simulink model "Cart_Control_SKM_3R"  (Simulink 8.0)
settings: Solver=FixedStepDiscrete  SolverMode=SingleTasking  StartTime=0  StopTime=6  FixedStep=dt  RelTol=1e-3  SampleTimeConstraint=Specified
InitFcn:
  | % Sampling Times %
  | dt0=0.001; dt1=0.01; samples=10;
  | D2R=pi/180;
undefined symbols (not defined in the file or in its folder): DiscIntNeverNeededParam, Volts
libraries: simulink_extras x4, speedgoatlib_IO311 x3, simulink x3, speedgoatlib_IO101 x2, xpclib x1

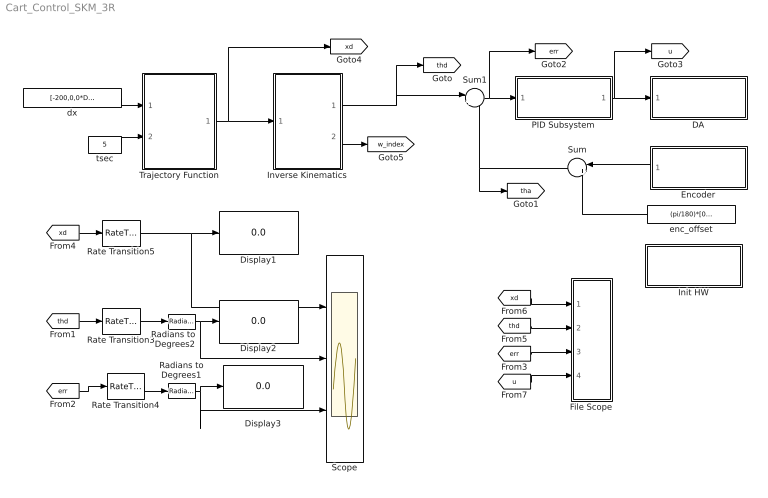
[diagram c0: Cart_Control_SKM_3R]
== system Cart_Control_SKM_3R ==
  DA : Subsystem  TreatAsAtomicUnit=on
  Display1 : Display
  Display2 : Display
  Display3 : Display
  Encoder : Subsystem  TreatAsAtomicUnit=on
  File Scope : Subsystem
  Init HW : Subsystem  TreatAsAtomicUnit=on
  Inverse Kinematics : MATLAB Function  TreatAsAtomicUnit=on
  PID Subsystem : Subsystem  TreatAsAtomicUnit=on
  Radians to Degrees1 : simulink_extras/Transformations/Radians to Degrees
  Radians to Degrees2 : simulink_extras/Transformations/Radians to Degrees
  Rate Transition3 : RateTransition  OutPortSampleTime=dt1
  Rate Transition4 : RateTransition  OutPortSampleTime=dt1
  Rate Transition5 : RateTransition  OutPortSampleTime=dt1
  Scope : Scope  NumInputPorts=3
  Sum : Sum  Inputs=|++
  Sum1 : Sum  Inputs=|+-
  Trajectory Function : MATLAB Function  TreatAsAtomicUnit=on
  dx : Constant  Value=[-200,0,0*D2R]'  SampleTime=dt0
  enc_offset : Constant  Value=(pi/180)*[0,90,0]'
  tsec : Constant  Value=5  SampleTime=dt0
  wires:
  Sum1/1 -> PID Subsystem/1(In1), [err]
  PID Subsystem/1(Out1) -> DA/1(In1), [u]
  Encoder/1(Out1) -> Sum/1
  enc_offset/1 -> Sum/2
  Sum/1 -> Sum1/2, [tha]
  [xd] -> File Scope/1(xd)
  [thd] -> File Scope/2(thd)
  [err] -> File Scope/3(err)
  [u] -> File Scope/4(u)
  dx/1 -> Trajectory Function/1(dx)
  tsec/1 -> Trajectory Function/2(tsec)
  Trajectory Function/1(xd) -> [xd], Inverse Kinematics/1(xd)
  Inverse Kinematics/1(thd) -> Sum1/1, [thd]
  [thd] -> Rate Transition3/1
  [err] -> Rate Transition4/1
  [xd] -> Rate Transition5/1
  Rate Transition5/1 -> Display1/1, Scope/1
  Rate Transition3/1 -> Radians to Degrees2/1
  Rate Transition4/1 -> Radians to Degrees1/1
  Radians to Degrees2/1 -> Display2/1, Scope/2
  Radians to Degrees1/1 -> Display3/1, Scope/3
  Inverse Kinematics/2(w_index) -> [w_index]

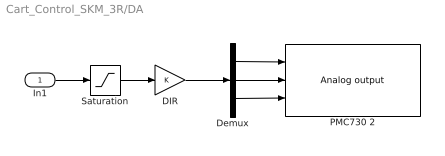
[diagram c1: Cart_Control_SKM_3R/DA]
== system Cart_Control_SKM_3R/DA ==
  In1 : Inport
  DIR : Gain
  Demux : Demux  Outputs=3
  PMC730 2 : speedgoatlib_IO101/Analog output  id=1  channel=[1,2,3]  reset=[1,1,1]  initValue=[0,0,0]  ts=dt0  pciSlot=-1
  Saturation : Saturate  UpperLimit=10  LowerLimit=-10
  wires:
  In1/1 -> Saturation/1
  Saturation/1 -> DIR/1
  DIR/1 -> Demux/1
  Demux/1 -> PMC730 2/1
  Demux/2 -> PMC730 2/2
  Demux/3 -> PMC730 2/3

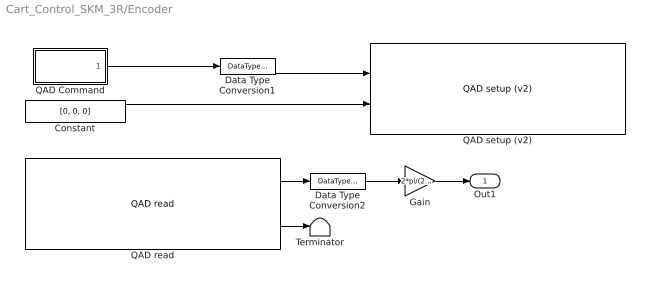
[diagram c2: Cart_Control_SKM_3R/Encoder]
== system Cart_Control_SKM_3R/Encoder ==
  Constant : Constant  Value=[0, 0, 0]  OutDataTypeStr=Inherit: Inherit via back propagation
  Data Type Conversion1 : DataTypeConversion  OutDataTypeStr=uint8
  Data Type Conversion2 : DataTypeConversion  OutDataTypeStr=double
  Gain : Gain  Gain=2*pi/(23*2000)
  QAD Command : MATLAB Function  TreatAsAtomicUnit=on
  QAD read : speedgoatlib_IO311/QAD/QAD read  id=1  chan=[1 2 3]  pciSlot=-1  ts=dt0
  QAD setup (v2) : speedgoatlib_IO311/QAD/QAD setup (v2)  id=1  chan=[1,2,3]  debounce=0  quadrature=4x  index=Ignore index input  special=Disabled (cycling counter)  steps=2000  ts=dt0  pciSlot=-1
  Terminator : Terminator
  Out1 : Outport
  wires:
  Gain/1 -> Out1/1
  Constant/1 -> QAD setup (v2)/2
  QAD read/2 -> Terminator/1
  QAD read/1 -> Data Type Conversion2/1
  QAD Command/1(y) -> Data Type Conversion1/1
  Data Type Conversion2/1 -> Gain/1
  Data Type Conversion1/1 -> QAD setup (v2)/1

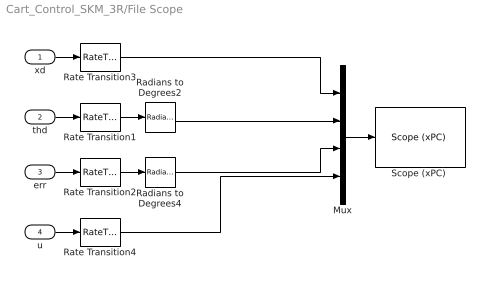
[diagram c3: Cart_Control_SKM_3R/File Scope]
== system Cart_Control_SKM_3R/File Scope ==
  xd : Inport
  thd : Inport  Port=2
  err : Inport  Port=3
  u : Inport  Port=4
  Mux : Mux
  Radians to Degrees2 : simulink_extras/Transformations/Radians to Degrees
  Radians to Degrees4 : simulink_extras/Transformations/Radians to Degrees
  Rate Transition{1..4} (4 alike) : RateTransition  OutPortSampleTime=dt1
  "Scope (xPC) " : xpclib/Misc./Scope (xPC)   scopeno=1  scopetype=File  autostart=on  viewmode=Graphical redraw  formatstr='%15.6f'  grid=on  ylimits=[0,0]  nosamples=100  noprepostsamples=0  interleave=1  triggermode=FreeRun  triggersignal=1  triggerlevel=0.0  triggerslope=Either  triggerscope=1  triggersample=0  filename=step2.dat  mode=Lazy  writesize=512  autorestart=on  dynamicfilemode=off  maxwritefilesize=512*1024^2
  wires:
  Radians to Degrees2/1 -> Mux/2
  Radians to Degrees4/1 -> Mux/3
  Rate Transition1/1 -> Radians to Degrees2/1
  Rate Transition2/1 -> Radians to Degrees4/1
  thd/1 -> Rate Transition1/1
  err/1 -> Rate Transition2/1
  Rate Transition3/1 -> Mux/1
  xd/1 -> Rate Transition3/1
  u/1 -> Rate Transition4/1
  Mux/1 -> "Scope (xPC) "/1
  Rate Transition4/1 -> Mux/4

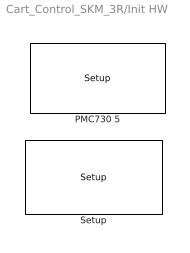
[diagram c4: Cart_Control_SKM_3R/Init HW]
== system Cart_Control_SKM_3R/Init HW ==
  PMC730 5 : speedgoatlib_IO101/Setup  group=Analog output setup  id=1  pciSlot=-1  adStartChannel=1  adNumChannel=1  adCoupling=Single-ended  adRange=-10 .. 10 Volts  adAcqMode=Standard  daChannel=[1,2,3]  daReset=[1,1,1]  daInitValue=[0,0,0]  lowerChannel=1  lowerDirection=Input  lowerDIDebounce=0  lowerDOReset=[1]  lowerDOInitValues=[0]  upperChannel=1  upperDirection=Output  upperDIDebounce=0  upperDOReset=0  upperDOInitValues=0
  Setup : speedgoatlib_IO311/Setup/Setup  group=Upper channel group setup  id=1  fpga1=speedgoat_IO311_default  pciSlot=-1  lowerDirection=[1 1 1 1 1 0 0 0 0 0 0 0 1 0 0 0]  lowerReset=[1]  lowerValue=[0]  upperDirection=[1 1 1 1 1 1 1 1 1 0 0 0 0 0 0 0]  upperReset=[1]  upperValue=[0]

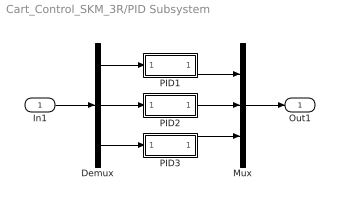
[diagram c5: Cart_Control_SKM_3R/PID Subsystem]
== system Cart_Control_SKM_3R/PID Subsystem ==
  In1 : Inport
  Demux : Demux  Outputs=3
  Mux : Mux  Inputs=3
  PID1 : Subsystem
  PID2 : Subsystem
  PID3 : Subsystem
  Out1 : Outport
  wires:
  In1/1 -> Demux/1
  Demux/1 -> PID1/1(In1)
  PID1/1(Out1) -> Mux/1
  Demux/2 -> PID2/1(In1)
  PID2/1(Out1) -> Mux/2
  Mux/1 -> Out1/1
  Demux/3 -> PID3/1(In1)
  PID3/1(Out1) -> Mux/3

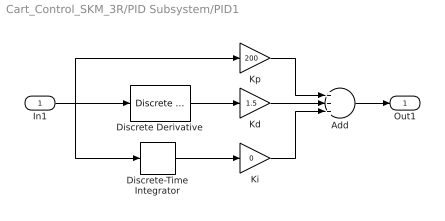
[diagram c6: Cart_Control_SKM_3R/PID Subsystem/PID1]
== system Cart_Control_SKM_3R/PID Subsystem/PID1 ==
  In1 : Inport
  Add : Sum  Inputs=+++
  Discrete Derivative : simulink/Discrete/Discrete Derivative  gainval=1.0  ICPrevScaledInput=0.0  InputProcessing=Inherited  OutMin=[]  OutMax=[]  OutDataType=fixdt(1, 16)  OutScaling=2^-10  DoSatur=off
  Discrete-Time Integrator : DiscreteIntegrator  SampleTime=dt0  ICPrevOutput=DiscIntNeverNeededParam  ICPrevScaledInput=DiscIntNeverNeededParam
  Kd : Gain  Gain=1.5
  Ki : Gain  Gain=0
  Kp : Gain  Gain=200
  Out1 : Outport
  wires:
  Discrete-Time Integrator/1 -> Ki/1
  Kp/1 -> Add/1
  Kd/1 -> Add/2
  Ki/1 -> Add/3
  Discrete Derivative/1 -> Kd/1
  Add/1 -> Out1/1
  In1/1 -> Kp/1, Discrete Derivative/1, Discrete-Time Integrator/1

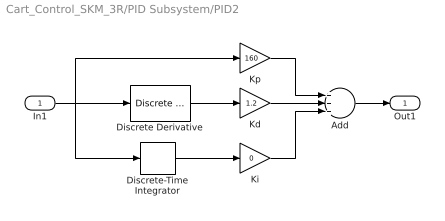
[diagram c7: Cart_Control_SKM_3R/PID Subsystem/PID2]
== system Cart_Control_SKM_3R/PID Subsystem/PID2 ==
  In1 : Inport
  Add : Sum  Inputs=+++
  Discrete Derivative : simulink/Discrete/Discrete Derivative  gainval=1.0  ICPrevScaledInput=0.0  InputProcessing=Inherited  OutMin=[]  OutMax=[]  OutDataType=fixdt(1, 16)  OutScaling=2^-10  DoSatur=off
  Discrete-Time Integrator : DiscreteIntegrator  SampleTime=dt0  ICPrevOutput=DiscIntNeverNeededParam  ICPrevScaledInput=DiscIntNeverNeededParam
  Kd : Gain  Gain=1.2
  Ki : Gain  Gain=0
  Kp : Gain  Gain=160
  Out1 : Outport
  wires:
  Discrete-Time Integrator/1 -> Ki/1
  Kp/1 -> Add/1
  Kd/1 -> Add/2
  Ki/1 -> Add/3
  Discrete Derivative/1 -> Kd/1
  Add/1 -> Out1/1
  In1/1 -> Kp/1, Discrete Derivative/1, Discrete-Time Integrator/1

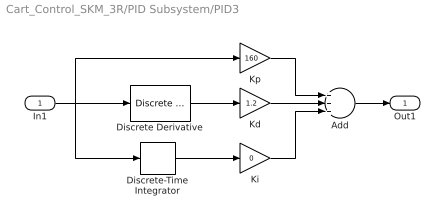
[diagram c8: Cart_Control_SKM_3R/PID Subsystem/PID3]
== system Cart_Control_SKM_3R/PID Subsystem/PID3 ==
  In1 : Inport
  Add : Sum  Inputs=+++
  Discrete Derivative : simulink/Discrete/Discrete Derivative  gainval=1.0  ICPrevScaledInput=0.0  InputProcessing=Inherited  OutMin=[]  OutMax=[]  OutDataType=fixdt(1, 16)  OutScaling=2^-10  DoSatur=off
  Discrete-Time Integrator : DiscreteIntegrator  SampleTime=dt0  ICPrevOutput=DiscIntNeverNeededParam  ICPrevScaledInput=DiscIntNeverNeededParam
  Kd : Gain  Gain=1.2
  Ki : Gain  Gain=0
  Kp : Gain  Gain=160
  Out1 : Outport
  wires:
  Discrete-Time Integrator/1 -> Ki/1
  Kp/1 -> Add/1
  Kd/1 -> Add/2
  Ki/1 -> Add/3
  Discrete Derivative/1 -> Kd/1
  Add/1 -> Out1/1
  In1/1 -> Kp/1, Discrete Derivative/1, Discrete-Time Integrator/1

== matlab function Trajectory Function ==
function xd = fcn(dx, tsec)

persistent index xd_p

MAX_CH=3;       % 3 Actuators %
dt=0.001;       % Step time is 10 msec %
a1=100; a2=70; a3=50;

% Initializing Variables %
if isempty(index), index=0; end
if isempty(xd_p), xd_p=zeros(MAX_CH,1); end
xd=zeros(MAX_CH,1);
x0=[a1,a2+a3, pi/2]';

tout=index*dt;
if index<(tsec/dt)
    [c] = coeff_3rd(x0, zeros(MAX_CH,1), x0+dx, zeros(MAX_CH,1), tsec);
    for ch=1:MAX_CH
        xd(ch,1)=c(ch,1)+c(ch,2)*tout+c(ch,3)*tout^2+c(ch,4)*tout^3;    
    end
    xd_p=xd;
else
    xd=xd_p;
end
index=index+1;

function [c] = coeff_3rd(sp, sv, ep, ev, tsec)
MAX_CH=3;
c=zeros(MAX_CH,4);
for ch=1:MAX_CH
    c(ch,1)=sp(ch,1);
    c(ch,2)=sv(ch,1);
    c(ch,3)=(3.0*(ep(ch,1)-sp(ch,1))-(2.0*sv(ch,1)+ev(ch,1))*tsec)/(tsec*tsec);
    c(ch,4)=(-2.0*(ep(ch,1)-sp(ch,1))+(sv(ch,1)+ev(ch,1))*tsec)/(tsec*tsec*tsec);
end

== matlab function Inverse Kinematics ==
function [thd,w_index]  = fcn(xd)

persistent index thd_p

% Initializing Variables %
if isempty(index), index=0; end
if isempty(thd_p), thd_p=(pi/180)*[0,90,0]'; end

w_index=1;  % In workspace %
a1=100; a2=70; a3=50;

qx=xd(1,1); qy=xd(2,1); phi=xd(3,1);

% (1) Calculate th2 %
px=qx-a3*cos(phi); py=qy-a3*sin(phi);
kapha=(px^2+py^2-a1^2-a2^2)/(2*a1*a2);
if abs(kapha)>1
    w_index=-1;  % Out of Workspace %
    kapha=1;
end
th2=+acos(kapha); % Elbow Down %
%th2=-acos(kapha); % Elbow Up %
 
% (2) Calculate th1 %
delta=a1^2+a2^2+2*a1*a2*cos(th2);
cth1=(px*(a1+a2*cos(th2))+py*a2*sin(th2))/delta;
sth1=(-px*a2*sin(th2)+py*(a1+a2*cos(th2)))/delta;
th1=atan2(sth1, cth1);
if th1<0, th1=th1+2*pi; end % 0<th<360 %

% (3) Calcuate th3 %
th3=phi-(th1+th2);

% (3) Check Joint Limits %
if th1<0 || th1>pi, w_index=-1; end
if th2<pi/6 || th2>5*pi/6, w_index=-1; end

% Result %
if w_index==1
    thd=[th1, th2, th3]';
else
    thd=thd_p;
end

% Save the current value %
thd_p=thd;

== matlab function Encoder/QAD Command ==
function y = fcn()

persistent index

if isempty(index), index=0; end

if index==0
    y=[1,1,1];      %  Reset %
else
    y = [0,0,0];
end

index=index+1;
